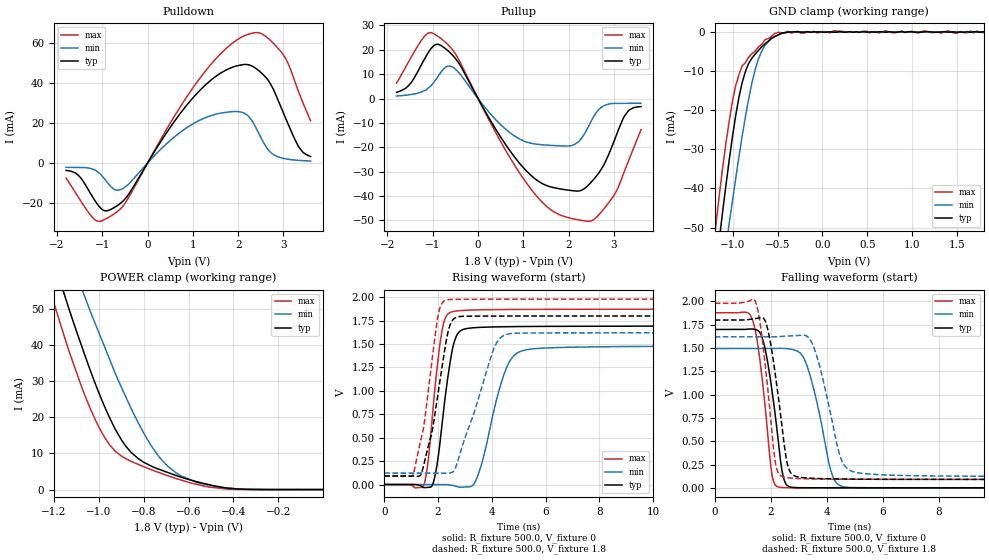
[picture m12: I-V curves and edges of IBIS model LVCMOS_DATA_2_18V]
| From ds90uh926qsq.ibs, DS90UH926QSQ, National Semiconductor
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[Model] LVCMOS_DATA_2_18V
Model_type 3-state
Enable Active-High
Vmeas = 0.9V
Cref = 0.0pF
Rref = 1.0e10
Vref = 0.0V
C_comp   2.75pF   2.32pF   3.18pF
[Voltage Range]   1.8V   1.62V   1.98V
[Temperature Range]   25.0   130.0   -40.0
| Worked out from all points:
|   slope of the pulldown table from 0 to 0.27 V, typ, clamps not added: 27.1 ohm
|   slope of the pullup table from 0 to 0.27 V, typ, clamps not added: 30.4 ohm
|   GND clamp passes 1 mA (typ) near -0.52 V on its own axis
|   POWER clamp passes 1 mA (typ) near -0.48 V on its own axis
|   rising waveform, R_fixture 500.0, V_fixture 0: 20-80 % time 453ps typ, 773ps min, 394ps max; typ from 0 V to 1.69 V
|   falling waveform, R_fixture 500.0, V_fixture 0: 20-80 % time 446ps typ, 639ps min, 398ps max; typ from 1.7 V to 0 V
|   rising waveform, R_fixture 500.0, V_fixture 1.8: 20-80 % time 600ps typ, 1.01ns min, 543ps max; typ from 0.09 V to 1.8 V
|   falling waveform, R_fixture 500.0, V_fixture 1.8: 20-80 % time 450ps typ, 668ps min, 390ps max; typ from 1.8 V to 0.09 V
[GND Clamp]
-1.8V     -191.5mA   -185.8mA   -190.4mA
-1.186V   -60.51mA   -74.1mA    -49.19mA
-1.148V   -52.87mA   -67.37mA   -41.47mA
-1.115V   -46.5mA    -61.8mA    -35.31mA
-1.038V   -32.65mA   -48.82mA   -22.64mA
-966.7mV  -21.44mA   -37.59mA   -13.74mA
-895.4mV  -13.06mA   -26.84mA   -8.701mA
-824.2mV  -8.131mA   -17.39mA   -6.503mA
-747.4mV  -5.603mA   -9.444mA   -4.828mA
-637.8mV  -3.007mA   -3.333mA   -1.937mA
-533.6mV  -1.207mA   -1.187mA   -419.4uA
1.796V    83.51uA    0A         -169.6uA
[POWER Clamp]
-1.8V     189.4mA    185.2mA    187.4mA
-1.219V   66.83mA    79.85mA    55.61mA
-1.202V   63.63mA    77.01mA    52.24mA
-1.148V   52.96mA    67.56mA    41.3mA
-1.06V    36.85mA    53.03mA    25.82mA
-966.7mV  21.93mA    38.4mA     13.74mA
-879mV    12mA       25.6mA     8.56mA
-769.3mV  6.604mA    12.45mA    5.591mA
-659.7mV  3.981mA    4.813mA    3.155mA
-550.1mV  1.973mA    1.699mA    1.249mA
-440.4mV  533.9uA    453uA      213.3uA
-1.827mV  614nA      -3.035uA   -1.983uA
[Pullup]
-1.8V     2.538mA    1.037mA    6.358mA
-1.148V   17.33mA    3.544mA    26.25mA
-818.7mV  21.77mA    10.8mA     24.61mA
-550.1mV  17.53mA    12.84mA    19.69mA
431.3mV   -13.81mA   -9.474mA   -15.36mA
1.034V    -29.07mA   -17.62mA   -33.76mA
1.577V    -36.13mA   -19.19mA   -45.24mA
2.18V     -37.98mA   -18.28mA   -49.66mA
2.509V    -34.11mA   -8.909mA   -50.17mA
2.942V    -20.37mA   -2.118mA   -41.34mA
3.271V    -6.252mA   -1.982mA   -27.99mA
3.6V      -3.326mA   -1.967mA   -12.77mA
[Pulldown]
-1.8V     -3.706mA   -2.144mA   -7.565mA
-1.477V   -7.386mA   -2.221mA   -18.93mA
-1.148V   -19.3mA    -3.654mA   -28.65mA
-928.3mV  -23.95mA   -8.523mA   -27.99mA
-659.7mV  -21.18mA   -13.63mA   -24.17mA
1.089V    34.77mA    20.69mA    40.36mA
1.906V    48.14mA    25.73mA    60.48mA
2.29V     48.68mA    21.64mA    64.81mA
2.668V    41.26mA    6.452mA    62.25mA
2.997V    25.16mA    2.328mA    54.13mA
3.326V    8.406mA    1.358mA    36.1mA
3.6V      3.243mA    998.1uA    21.19mA
[Rising Waveform]
R_fixture=500.0
V_fixture=0
V_fixture_min=0
V_fixture_max=0
0s        22.29nV    566nV      518.4pV
1.45ns    -32.01mV   543.3nV    -21.05mV
1.6ns     -31.06mV   -564.4nV   185.1mV
1.8ns     -1.455mV   -7.612uV   769.9mV
2.2ns     780.2mV    108.1uV    1.719V
2.7ns     1.598V     -22.09mV   1.854V
3.45ns    1.677V     73.29mV    1.865V
4.65ns    1.686V     1.311V     1.869V
5.5ns     1.688V     1.448V     1.871V
49.98ns   1.694V     1.485V     1.874V
[Falling Waveform]
R_fixture=500.0
V_fixture=0
V_fixture_min=0
V_fixture_max=0
0s        1.699V     1.495V     1.878V
1.35ns    1.704V     1.495V     1.801V
1.8ns     1.49V      1.495V     875.7mV
2.05ns    1.033V     1.495V     126.6mV
2.35ns    287.5mV    1.497V     4.603mV
2.55ns    36.45mV    1.494V     1.666mV
3.2ns     1.223mV    1.38V      572.6uV
4.2ns     455.1uV    131.9mV    260.9uV
4.7ns     321.5uV    6.901mV    188.3uV
49.98ns   4.563uV    11.99uV    2.908uV
[Rising Waveform]
R_fixture=500.0
V_fixture=1.8
V_fixture_min=1.62
V_fixture_max=1.98
0s        90.38mV    122.1mV    90.85mV
1.05ns    90.43mV    122.1mV    92.27mV
1.35ns    97.63mV    122.1mV    465.5mV
1.75ns    532.2mV    122.1mV    1.269V
2ns       975.4mV    122.1mV    1.804V
2.35ns    1.605V     121mV      1.973V
2.65ns    1.782V     177.2mV    1.978V
4.1ns     1.799V     1.47V      1.98V
4.7ns     1.8V       1.612V     1.98V
49.98ns   1.8V       1.62V      1.98V
[Falling Waveform]
R_fixture=500.0
V_fixture=1.8
V_fixture_min=1.62
V_fixture_max=1.98
0s        1.8V       1.62V      1.98V
1.4ns     1.813V     1.62V      2.023V
1.6ns     1.824V     1.62V      1.804V
1.8ns     1.792V     1.62V      1.325V
2.2ns     1.134V     1.622V     214.8mV
2.6ns     247.4mV    1.628V     108.2mV
3.45ns    103mV      1.567V     96.11mV
4.5ns     94.99mV    319mV      92.87mV
5.3ns     92.82mV    153.5mV    91.97mV
49.98ns   90.38mV    122.1mV    90.86mV
[Ramp]
R_load = 500.0
dV/dt_r   1.016429E0/4.5E-10   8.91002E-1/8E-10   1.124492E0/4E-10
dV/dt_f   1.025772E0/4.5E-10   8.987499E-1/6.5E-10   1.133484E0/4E-10
